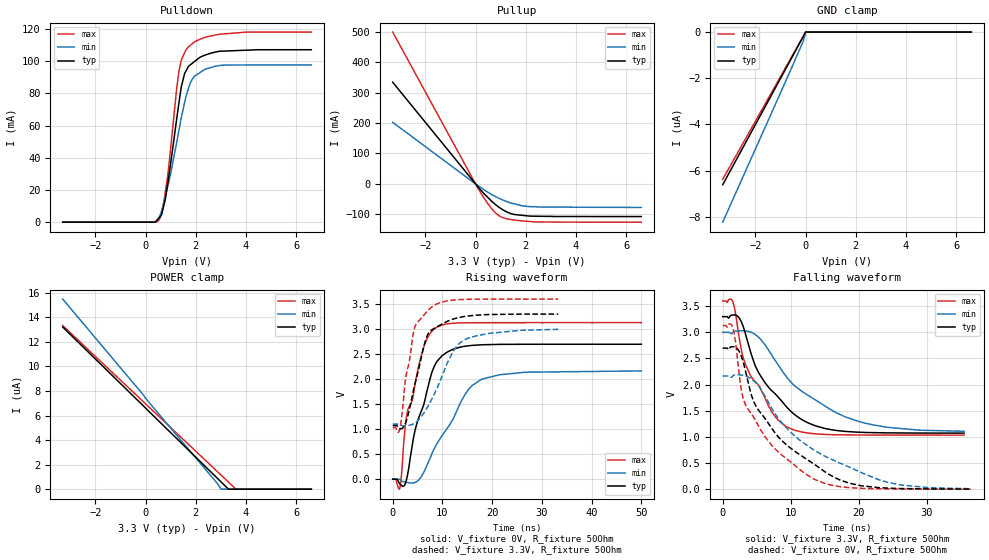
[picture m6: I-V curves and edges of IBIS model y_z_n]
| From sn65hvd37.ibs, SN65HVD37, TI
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[Model]   y_z_n
Model_type   3-state
Polarity   Non-Inverting
Vmeas = 1.65
Vref = 1.65
Cref = 50pF
Rref = 50
|   typ   min   max
|   (nom PVT)   (fast PVT)   (slow PVT)
|C_Comp from frequency method(F=10MHz)
|C_comp   1.308e-10   8.009e-11   1.915e-10
|ON state
|C_comp   1.308e-10   8.009e-11   1.915e-10
|OFF state
|C_comp   1.822e-11   1.815e-11   1.847e-11
|C_Comp from L-C Tank method(L=1nH)
|Resonant Frequency(Hz)   1.070e+09   1.100e+09   1.068e+09
C_comp   1.455e-11   1.371e-11   1.548e-11
|ON state
|Resonant Frequency(Hz)   1.070e+09   1.100e+09   1.068e+09
|C_comp   2.215e-11   2.095e-11   2.221e-11
|OFF state
|Resonant Frequency(Hz)   1.490e+09   1.540e+09   1.450e+09
|C_comp   1.142e-11   1.069e-11   1.206e-11
| Where nom  PVT is Nominal Process, 3.3V, 27C
|   Fast PVT is Strong Process,  3.6V, -40C
|   Slow PVT is Weak Process,   3V, 125C
[Voltage Range]   3.3   3   3.6
|Ambient Temperature   25   85   -40
|Junction Temperature
[Temperature Range]   27   125   -40
[Pullup Reference]   3.3   3   3.6
[Pulldown Reference]   0   0   0
[Power Clamp Reference]   3.3   3   3.6
[GND Clamp Reference]   0   0   0
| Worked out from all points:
|   slope of the pulldown table from 0 to 0.495 V, typ, clamps not added: 253 ohm
|   slope of the pullup table from 0 to 0.495 V, typ, clamps not added: 11 ohm
|   falling waveform, V_fixture 3.3V, R_fixture 50Ohm: 20-80 % time 6.2ns typ, 9.43ns min, 4.72ns max; typ from 3.3 V to 1.07 V
|   rising waveform, V_fixture 0V, R_fixture 50Ohm: 20-80 % time 4.26ns typ, 7.25ns min, 3.7ns max; typ from 0 V to 2.7 V
|   rising waveform, V_fixture 3.3V, R_fixture 50Ohm: 20-80 % time 3.27ns typ, 5.36ns min, 2.52ns max; typ from 1.07 V to 3.3 V
|   falling waveform, V_fixture 0V, R_fixture 50Ohm: 20-80 % time 9.18ns typ, 11.9ns min, 6.78ns max; typ from 2.7 V to 0.003 V
[Pulldown]
|   Voltage   I(typ)   I(min)   I(max)
-3.3V     -1.596nA   -10.33nA   -384.2pA
326.7mV   33.39uA    104.4uA    55.43uA
540mV     2.779mA    2.8mA      1.538mA
633.6mV   4.495mA    6.841mA    5.548mA
860.4mV   21.76mA    20.65mA    26.43mA
1.242V    64.5mA     49.71mA    83.62mA
1.332V    74.42mA    57.38mA    94mA
1.554V    92.36mA    74.35mA    105.1mA
1.761V    97.45mA    85.72mA    109.5mA
1.912V    99.29mA    89.91mA    111.5mA
3.074V    106.2mA    97.52mA    116.9mA
6.6V      107.1mA    97.67mA    118mA
[GND Clamp]
|   Voltage   I(typ)   I(min)   I(max)
-3.3V     -6.611uA   -8.231uA   -6.374uA
-171mV    -350.3nA   -590.2nA   -330.9nA
-69mV     -145.4nA   -310.2nA   -134nA
-24mV     -52.22nA   -125nA     -46.97nA
-3.3mV    0A         0A         0A
6.6V      0A         0A         0A
[Pullup]
|   Voltage   I(typ)   I(min)   I(max)
-3.3V     333.9mA    202.1mA    498.5mA
82.8mV    -8.117mA   -4.816mA   -12.03mA
478.8mV   -43.63mA   -26.58mA   -63.63mA
648mV     -57.42mA   -35.04mA   -81.84mA
885.6mV   -73.74mA   -45.37mA   -101.5mA
1.062V    -83.72mA   -52.1mA    -110.1mA
1.403V    -97.21mA   -62.39mA   -116.8mA
1.836V    -102.9mA   -71.53mA   -121.2mA
2.168V    -105.7mA   -74.55mA   -123.3mA
6.6V      -107.2mA   -77.14mA   -125.6mA
[POWER Clamp]
|   Voltage   I(typ)   I(min)   I(max)
-3.3V     13.22uA    15.49uA    13.33uA
2.844V    915.9nA    494nA      1.459uA
3V        603.9nA    0A         1.158uA
3.297V    0A         0A         585.2nA
3.596V    0A         0A         0A
6.6V      0A         0A         0A
[Ramp]
R_load = 50
|   typ   min   max
dV/dt_r   1.61828/4.25257e-09   1.29837/7.23356e-09   1.87722/3.69767e-09
dV/dt_f   1.33667/6.22071e-09   1.13863/9.49246e-09   1.53953/4.72642e-09
[Falling Waveform]
V_fixture = 3.3V
V_fixture_min = 3V
V_fixture_max = 3.6V
R_fixture = 50Ohm
|   Time   V(typ)   V(min)   V(max)
0s        3.3V       3V         3.6V
1.5ns     3.331V     3.001V     3.579V
2.44ns    3.271V     3.029V     2.883V
3.29ns    2.995V     3.028V     2.404V
5.23ns    2.24V      2.913V     1.997V
7.68ns    1.828V     2.471V     1.394V
9.53ns    1.554V     2.123V     1.187V
13.67ns   1.211V     1.706V     1.059V
19.97ns   1.09V      1.296V     1.037V
35.49ns   1.073V     1.108V     1.034V
[Rising Waveform]
V_fixture = 0V
V_fixture_min = 0V
V_fixture_max = 0V
R_fixture = 50Ohm
|   Time   V(typ)   V(min)   V(max)
0s        25.24nV    80.59nV    25.61nV
1.45ns    -94.48mV   -5.371mV   -167.6mV
2.51ns    -95.05mV   -58.12mV   1.044V
2.95ns    69.63mV    -66.26mV   1.353V
4.59ns    1.014V     -59.98mV   1.951V
6.19ns    1.473V     127.9mV    2.621V
8.71ns    2.323V     677.3mV    3.028V
15.26ns   2.667V     1.794V     3.127V
18.14ns   2.687V     2.006V     3.128V
50ns      2.697V     2.164V     3.129V
[Rising Waveform]
V_fixture = 3.3V
V_fixture_min = 3V
V_fixture_max = 3.6V
R_fixture = 50Ohm
|   Time   V(typ)   V(min)   V(max)
0s        1.071V     1.101V     1.032V
1.45ns    1.009V     1.093V     1.011V
2.62ns    1.132V     1.069V     2.03V
4.51ns    1.919V     1.127V     3.059V
6.65ns    2.792V     1.382V     3.324V
7.97ns    2.992V     1.622V     3.449V
12.11ns   3.198V     2.546V     3.579V
14.14ns   3.247V     2.769V     3.592V
19.54ns   3.291V     2.915V     3.599V
33.28ns   3.3V       2.995V     3.6V
[Falling Waveform]
V_fixture = 0V
V_fixture_min = 0V
V_fixture_max = 0V
R_fixture = 50Ohm
|   Time   V(typ)   V(min)   V(max)
0s        2.698V     2.165V     3.13V
1.52ns    2.725V     2.17V      3.075V
2.77ns    2.53V      2.183V     1.866V
3.36ns    2.258V     2.166V     1.614V
5.22ns    1.519V     1.982V     1.222V
8.25ns    990.1mV    1.342V     702.6mV
12.05ns   598.7mV    870.4mV    303.8mV
20.14ns   72.2mV     332.9mV    18.84mV
26.14ns   13.52mV    82.19mV    4.767mV
36.56ns   2.854mV    9.122mV    1.513mV
